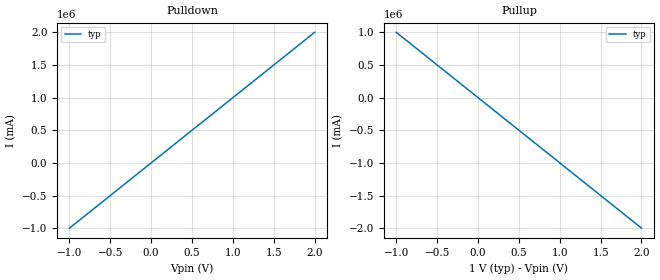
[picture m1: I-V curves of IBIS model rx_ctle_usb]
[IBIS Ver]   5.0
[File Name]  rx_usb_ctle.ibs
[File Rev]   1.0
[Component]  lvpe502a
[Manufacturer] Texas Instruments Incorporated
[Package]
R_pkg  0.0   NA   NA
L_pkg  0.0   NA   NA
C_pkg  0.0   NA   NA
[Pin]   signal_name   model_name   R_pin L_pin  C_pin
2p   Rx_p   rx_ctle_usb
2n   Rx_n   rx_ctle_usb
[Diff_Pin] inv_pin vdiff tdelay_typ tdelay_min tdelay_max
2p   2n   NA   NA   NA   NA
| Models and submodels in the file (1): rx_ctle_usb (Input)
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[Model] rx_ctle_usb
Model_type Input
C_comp 0p 0p 0p
Vinl = 0.3
Vinh = 0.7
[Temperature_Range] 25 125 0
[Voltage Range] 1.0 1.0 1.0
[Algorithmic Model]
Executable Windows_VisualC++ExpressEdition9.0.30729_32 rx_usb_ctle.dll rx_usb_ctle.ami
[End Algorithmic Model]
[Ramp]
|   typ   min   max
dV/dt_r   0.8/1.0ps   NA   NA
dV/dt_f   0.8/1.0ps   NA   NA
R_load = 0.001ohm
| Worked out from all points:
|   slope of the pulldown table from 0 to 0.15 V, typ, clamps not added: 1 mohm
|   slope of the pullup table from 0 to 0.15 V, typ, clamps not added: 1 mohm
[Pulldown]
|Voltage I(typ)   I(min)   I(max)
-1V       -1kA       NA         NA
0V        0A         NA         NA
2V        2kA        NA         NA
[Pullup]
-1V       1kA        NA         NA
0V        0A         NA         NA
2V        -2kA       NA         NA
[GND Clamp]
-1V       0A         0A         0A
0V        0A         0A         0A
2V        0A         0A         0A
[Power Clamp]
-1V       0A         0A         0A
0V        0A         0A         0A
2V        0A         0A         0A
